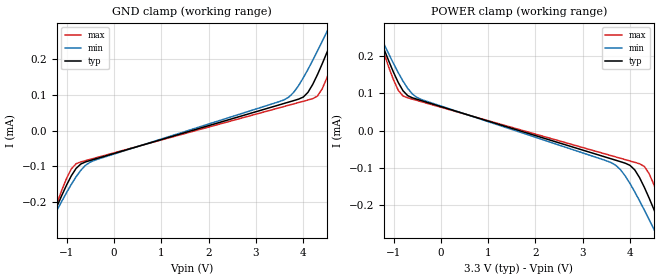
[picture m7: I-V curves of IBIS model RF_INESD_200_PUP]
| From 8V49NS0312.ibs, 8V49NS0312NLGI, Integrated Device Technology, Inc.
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[Model]   RF_INESD_200_PUP
Model_type   Input
Polarity   Non-Inverting
Vinl = 0.8V
Vinh = 2.0V
|   typ   min   max
C_comp   2pF   1.5pF   2.5pF
|   typ   min   max
[Voltage range]   3.3V   3.135V   3.465V
[GND_clamp]
|Voltage   I (typ)   I (min)   I (max)
|Note, modeling breaks down at 250mA and above.  This is well beyond the functional   |
|operating range of the device.  Should this scenario occur, catastrophic failure and   |
|possible damage to the device and/or board is of higher concern than the I-V curve   |
|behavior.  The IBIS checker will flag currents in excess of 10A with warnings.  Lines   |
|with currents in excess of 0.35 A have been commented out.  The points still remain|
|available to the user if the user desires to use them.   |
-3.3V     -908.7uA   -784.4uA   -1.041mA
-1.5V     -304.7uA   -297.8uA   -314.5uA
-1.4V     -272.6uA   -271.8uA   -275.9uA
-800mV    -105.4uA   -128.7uA   -92.51uA
-400mV    -79.52uA   -82.49uA   -76.62uA
3.6V      75.64uA    85.73uA    67.09uA
4.1V      106.4uA    170.2uA    85.06uA
4.3V      155.5uA    221.4uA    95.9uA
4.6V      249.8uA    302.8uA    181.7uA
4.7V      283.2uA    330.6uA    219.4uA
4.9V      351.4uA    386.9uA    298.3uA
6.6V      955.6uA    880.6uA    1.012mA
[Power_clamp]
|Voltage   I (typ)   I (min)   I (max)
|Note, modeling breaks down at 250mA and above.  This is well beyond the functional   |
|operating range of the device.  Should this scenario occur, catastrophic failure and   |
|possible damage to the device and/or board is of higher concern than the I-V curve   |
|behavior.  The IBIS checker will flag currents in excess of 10A with warnings.  Lines   |
|with currents in excess of 0.35 A have been commented out.  The points still remain|
|available to the user if the user desires to use them.   |
-3.3V     955.5uA    832.1uA    1.083mA
-1.4V     283.2uA    284.8uA    284.3uA
-1V       155.5uA    178.9uA    135uA
-800mV    106.4uA    132.1uA    92.33uA
-400mV    79.52uA    82.44uA    76.62uA
3.7V      -79.52uA   -93.18uA   -70.69uA
4V        -93.23uA   -142.1uA   -81.47uA
4.3V      -151.5uA   -212.3uA   -95.93uA
4.6V      -240.9uA   -288.7uA   -177.5uA
4.7V      -272.6uA   -314.8uA   -213.6uA
4.9V      -337.2uA   -367.5uA   -289.4uA
6.6V      -908.7uA   -829.8uA   -973.2uA
